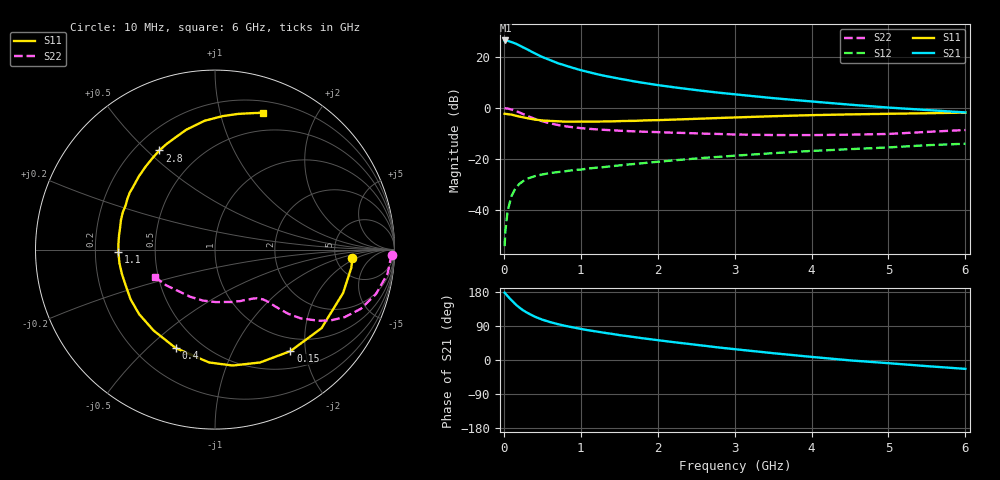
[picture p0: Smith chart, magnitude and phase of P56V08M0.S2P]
! SIEMENS Small Signal Semiconductors
! BFP183
! Si NPN RF Bipolar Junction Transistor in SOT143
! VCE = 6 V  IC = 8 mA
! Common Emitter S-Parameters:  March  1996
# GHz  S  MA  R  50
!  f  S11  S21  S12  S22
! GHz  MAG  ANG  MAG  ANG  MAG  ANG  MAG  ANG
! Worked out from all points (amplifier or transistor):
!   36 points, 10 MHz to 6 GHz, reference 50 ohm
!   highest |S21| = 26.6 dB at 20 MHz (marker M1)
!   |S21| within 3 dB of that: start of sweep to 269 MHz
!   unconditionally stable (mu >= 1): 1.346 GHz to 5.635 GHz
!   at 250 MHz: K = 0.27, MSG = 26.3 dB, |S12| = -28.8 dB
!   at 1.4 GHz: K = 1.02, MAG = 16.8 dB, |S12| = -23.0 dB
!   at 6 GHz: K = 0.95, MSG = 6.2 dB, |S12| = -14.1 dB
!   lowest NFmin = 1.30 dB at 450 MHz
!   S11 on the Smith chart (normalised r, x): 10 MHz: 7.17, -1.67; 150 MHz: 0.77, -1.72; 400 MHz: 0.36, -0.61; 1.1 GHz: 0.30, -0.01; 2.8 GHz: 0.30, +0.55; 6 GHz: 0.31, +1.37
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0.01  0.7666 -3.6  21.08 177.6  0.0019 78.4  0.9877 -1.6
0.02  0.7664 -7.5  21.26 175.5  0.0038 82.8  0.9796 -3.2
0.05  0.7535 -18.7  20.86 168.3  0.0096 82.2  0.9706 -8.0
0.1  0.7375 -36.4  19.72 157.6  0.0184 72.5  0.9299 -15.5
0.15  0.7047 -53.4  18.54 147.3  0.026 64.4  0.8768 -22.1
0.2  0.6773 -68.2  17.07 138.7  0.0317 58.9  0.8159 -27.4
0.25  0.6534 -81.3  15.54 131.2  0.0362 54.0  0.7569 -31.4
0.3  0.6297 -93.0  14.29 125.1  0.0402 50.4  0.6999 -34.5
0.4  0.5907 -111.7  11.92 114.5  0.0453 45.2  0.6104 -38.8
0.5  0.5659 -127.3  10.05 106.5  0.049 41.5  0.5463 -41.1
0.6  0.5549 -139.6  8.751 100.1  0.0522 39.8  0.498 -42.4
0.7  0.5458 -149.5  7.614 94.8  0.0545 38.7  0.4616 -43.3
0.9  0.5362 -165.2  6.127 86.1  0.0595 38.1  0.4156 -44.5
1.1  0.5383 -178.4  5.073 78.4  0.0643 38.3  0.3882 -45.9
1.3  0.5406 171.5  4.31 72.0  0.0685 38.5  0.3702 -47.7
1.6  0.5542 157.9  3.539 63.1  0.0765 39.1  0.3509 -50.9
2.2  0.5881 136.3  2.562 47.3  0.0926 38.9  0.3249 -60.1
2.8  0.6338 119.3  1.989 32.9  0.1091 36.6  0.3069 -72.1
3.5  0.6868 103.5  1.557 18.0  0.1286 33.6  0.2925 -88.9
4.5  0.7451 86.7  1.158 -1.0  0.1543 27.0  0.2971 -117.8
5.5  0.786 75.2  0.909 -16.2  0.1844 21.0  0.3368 -143.7
6  0.8089 70.5  0.815 -23.4  0.1974 16.9  0.3676 -155.4
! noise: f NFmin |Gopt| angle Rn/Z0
0.45  1.3  0.17  43  0.21
0.9  1.35  0.21  115  0.2
1.8  2.05  0.33  -177  0.14
